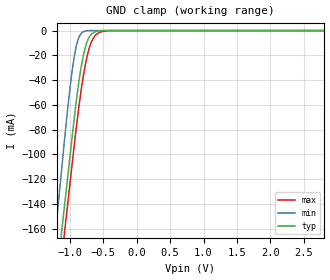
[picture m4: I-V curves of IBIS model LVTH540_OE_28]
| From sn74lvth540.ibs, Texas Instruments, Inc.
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[Model]   LVTH540_OE_28
Model_type  Input
Vinl = 0.8
Vinh = 2.0
| variable   typ   min   max
C_comp   1.77pF   1.42pF   2.20pF
[Temperature Range]   40   -40   100
| Ambient temperature   25   -40   85
[Voltage range]   2.8   2.7   2.9
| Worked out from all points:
|   GND clamp passes 1 mA (typ) near -0.62 V on its own axis
[GND Clamp]
| LVTH540_OE_28
|   Voltage   I(typ)   I(min)   I(max)
-5.5V     -2.407A    -2.647A    -2.408A
-1.22V    -209.3mA   -166mA     -230.3mA
-1.205V   -202mA     -157.5mA   -223mA
-1.125V   -163.1mA   -113mA     -184.4mA
-1.075V   -138.8mA   -85.24mA   -160.3mA
-975mV    -90.17mA   -36.12mA   -112.1mA
-900mV    -55.28mA   -11.44mA   -76.59mA
-800mV    -20.27mA   -984.6uA   -37mA
-675mV    -2.699mA   -6.758uA   -8.774mA
-575mV    -336.8uA   -57.38nA   -2.013mA
-425mV    -3.297uA   -110.8pA   -103uA
2.8V      13.7pA     7.338pA    757.3pA
